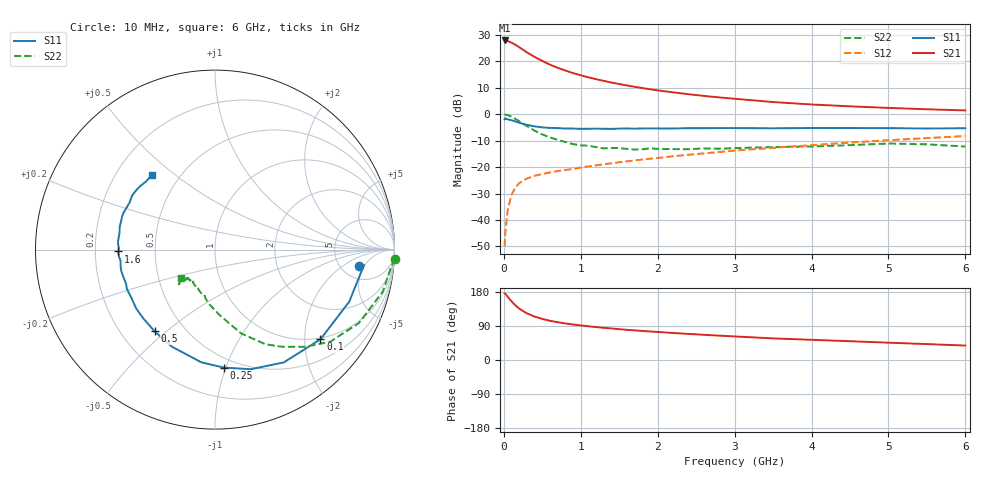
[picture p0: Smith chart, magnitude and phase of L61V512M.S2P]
!  INFINEON TECHNOLOGIES Small Signal Semiconductors
! BFR380L3 , Si-NPN RF-Transistor in TSLP-3-1
!  Vce=1.5 V,  Ic=12.5 mA
! Common Emitter S-Parameters:  07. March 2005
#  GHz  S  MA  R  50
! f  S11  S21  S12  S22
! GHz  Mag  Ang  Mag  Ang  Mag  Ang  Mag  Ang
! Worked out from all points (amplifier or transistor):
!   36 points, 10 MHz to 6 GHz, reference 50 ohm
!   highest |S21| = 28.0 dB at 10 MHz (marker M1)
!   |S21| within 3 dB of that: start of sweep to 222.6 MHz
!   unconditionally stable (mu >= 1): 2.037 GHz to 4.892 GHz
!   at 250 MHz: K = 0.29, MSG = 24.7 dB, |S12| = -25.1 dB
!   at 1.4 GHz: K = 0.91, MSG = 15.3 dB, |S12| = -18.5 dB
!   at 6 GHz: K = 0.98, MSG = 4.8 dB, |S12| = -8.2 dB
!   S11 on the Smith chart (normalised r, x): 10 MHz: 7.20, -3.87; 100 MHz: 0.96, -2.38; 250 MHz: 0.42, -0.98; 500 MHz: 0.34, -0.46; 1.6 GHz: 0.30, -0.01; 6 GHz: 0.35, +0.42
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0.01  0.806 -6.7  24.99 175.5  0.0032 84.6  1.002 -2.9
0.02  0.8347 -5.9  24.86 174.9  0.006 86.0  0.9855 -5.8
0.05  0.8023 -21.2  24.36 166.8  0.0154 79.4  0.964 -14.0
0.1  0.7713 -40.4  22.71 154.9  0.03 71.9  0.9005 -27.0
0.15  0.7362 -58.6  20.73 144.3  0.0411 63.4  0.8223 -38.6
0.2  0.6957 -73.3  18.59 135.8  0.0498 58.2  0.7395 -47.1
0.25  0.6591 -85.8  16.66 129.0  0.0558 53.8  0.6574 -55.4
0.3  0.6325 -96.9  14.88 123.2  0.061 51.3  0.5981 -61.9
0.4  0.5918 -113.9  12.19 114.5  0.0687 48.1  0.4891 -72.7
0.5  0.5661 -126.4  10.22 108.4  0.0742 46.9  0.4159 -79.3
0.6  0.5537 -136.2  8.696 103.4  0.0796 46.5  0.3665 -85.8
0.7  0.5483 -143.2  7.605 99.7  0.0842 47.2  0.3277 -91.8
0.9  0.5379 -155.9  6.024 93.6  0.0925 48.9  0.2732 -101.5
1.1  0.5327 -163.6  5.012 88.9  0.1033 50.9  0.2545 -107.9
1.4  0.5299 -173.1  3.99 83.3  0.1183 53.3  0.23 -115.7
1.6  0.5393 -178.9  3.516 79.6  0.1289 54.4  0.2213 -123.6
2.2  0.5405 169.7  2.605 71.3  0.161 57.6  0.2199 -128.3
2.8  0.5498 160.1  2.089 64.3  0.1936 59.3  0.2235 -135.3
3.5  0.5434 151.0  1.707 57.0  0.2319 58.8  0.2403 -135.7
4.5  0.5503 144.2  1.416 49.6  0.292 58.8  0.2612 -136.2
5.5  0.5397 135.3  1.247 42.0  0.3552 56.2  0.2704 -137.0
6  0.5458 130.0  1.184 38.1  0.3882 54.4  0.2459 -139.7
